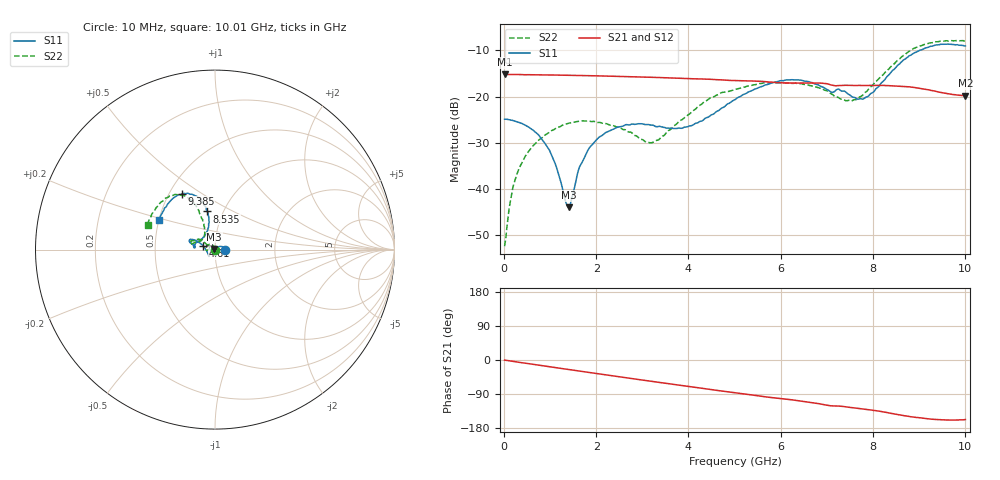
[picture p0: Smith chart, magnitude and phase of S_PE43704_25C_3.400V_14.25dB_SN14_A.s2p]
! Device ID: PE43704
! Dir: z:\PE43704\PE43704_Char_1_20130516\PE43704\AMB\3p400V\14p25dB
! Serial: 14
! Insertion: A
! Impedance: 50 ohm
! Temp: Amb
! VDD: 3.400V
! Attenuation Step: 14.25dB
! IDD: 1.140073e-01mA
#  Hz  S  RI  R  50
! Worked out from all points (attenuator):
!   401 points, 10 MHz to 10.01 GHz, reference 50 ohm
!   highest |S21| = -15.20 dB at 10 MHz (marker M1); lowest = -19.8 dB at 10.01 GHz (marker M2)
!   lowest |S11| = -43.9 dB at 1.41 GHz (marker M3), VSWR 1.01, Z = 49.5 + j0.404 ohm
!   |S11| at or under -10 dB: start of sweep to 9.019 GHz
!   |S22| runs from -52.3 to -7.9 dB; largest |S21 - S12| = 0.0011
!   S11 on the Smith chart (normalised r, x): 10 MHz: 1.12, +0.00; 4.61 GHz: 0.88, +0.04; 8.535 GHz: 0.84, +0.37; 9.385 GHz: 0.58, +0.41; 10.01 GHz: 0.50, +0.19
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1e7  0.0569 0.000162  0.1737 -0.000624  0.1738 -0.000585  -0.00236 0.000497
2.1e8  0.0543 0.00655  0.1728 -0.0118  0.1728 -0.0118  -0.00304 0.0109
4.35e8  0.0481 0.013  0.1706 -0.0239  0.1709 -0.0239  -0.00758 0.0202
9.6e8  0.0219 0.0167  0.1636 -0.0508  0.1635 -0.0507  -0.028 0.0292
1.335e9  -0.000791 0.00726  0.1555 -0.0689  0.1555 -0.0689  -0.0446 0.023
1.41e9  -0.00488 0.00408  0.1536 -0.0724  0.1536 -0.0723  -0.0473 0.0209
1.685e9  -0.0179 -0.00689  0.1462 -0.0847  0.1463 -0.0846  -0.0535 0.0118
1.885e9  -0.0251 -0.0152  0.1401 -0.093  0.1401 -0.0929  -0.0535 0.00511
2.26e9  -0.031 -0.0283  0.1273 -0.1073  0.1274 -0.1072  -0.0499 -0.00248
3.11e9  -0.0344 -0.0361  0.0936 -0.1325  0.0938 -0.1324  -0.0316 0.00542
3.36e9  -0.0361 -0.0312  0.0827 -0.1378  0.0828 -0.1376  -0.0317 0.0132
4.01e9  -0.0476 -0.00629  0.0536 -0.1471  0.0537 -0.1471  -0.0537 0.0349
4.61e9  -0.0661 0.02  0.0264 -0.1502  0.0267 -0.1501  -0.0871 0.0562
5.01e9  -0.085 0.0371  0.00983 -0.1488  0.00993 -0.1489  -0.1074 0.052
5.96e9  -0.1349 0.0574  -0.0275 -0.1387  -0.0271 -0.1389  -0.1347 0.0402
6.685e9  -0.1367 0.0368  -0.0535 -0.1295  -0.0537 -0.1293  -0.1263 0.0332
7.585e9  -0.0817 0.0546  -0.0782 -0.1065  -0.0783 -0.1062  -0.0636 0.0668
7.86e9  -0.0556 0.082  -0.0854 -0.1006  -0.0853 -0.1008  -0.0573 0.0974
8.36e9  -0.0344 0.1705  -0.1003 -0.0845  -0.1001 -0.0848  -0.077 0.1865
8.535e9  -0.0432 0.2125  -0.1043 -0.0768  -0.1038 -0.0773  -0.0977 0.2257
9.385e9  -0.186 0.3099  -0.1045 -0.044  -0.1047 -0.0437  -0.2588 0.2935
1.001e10  -0.3112 0.1668  -0.0945 -0.0399  -0.0954 -0.0397  -0.3757 0.1364
